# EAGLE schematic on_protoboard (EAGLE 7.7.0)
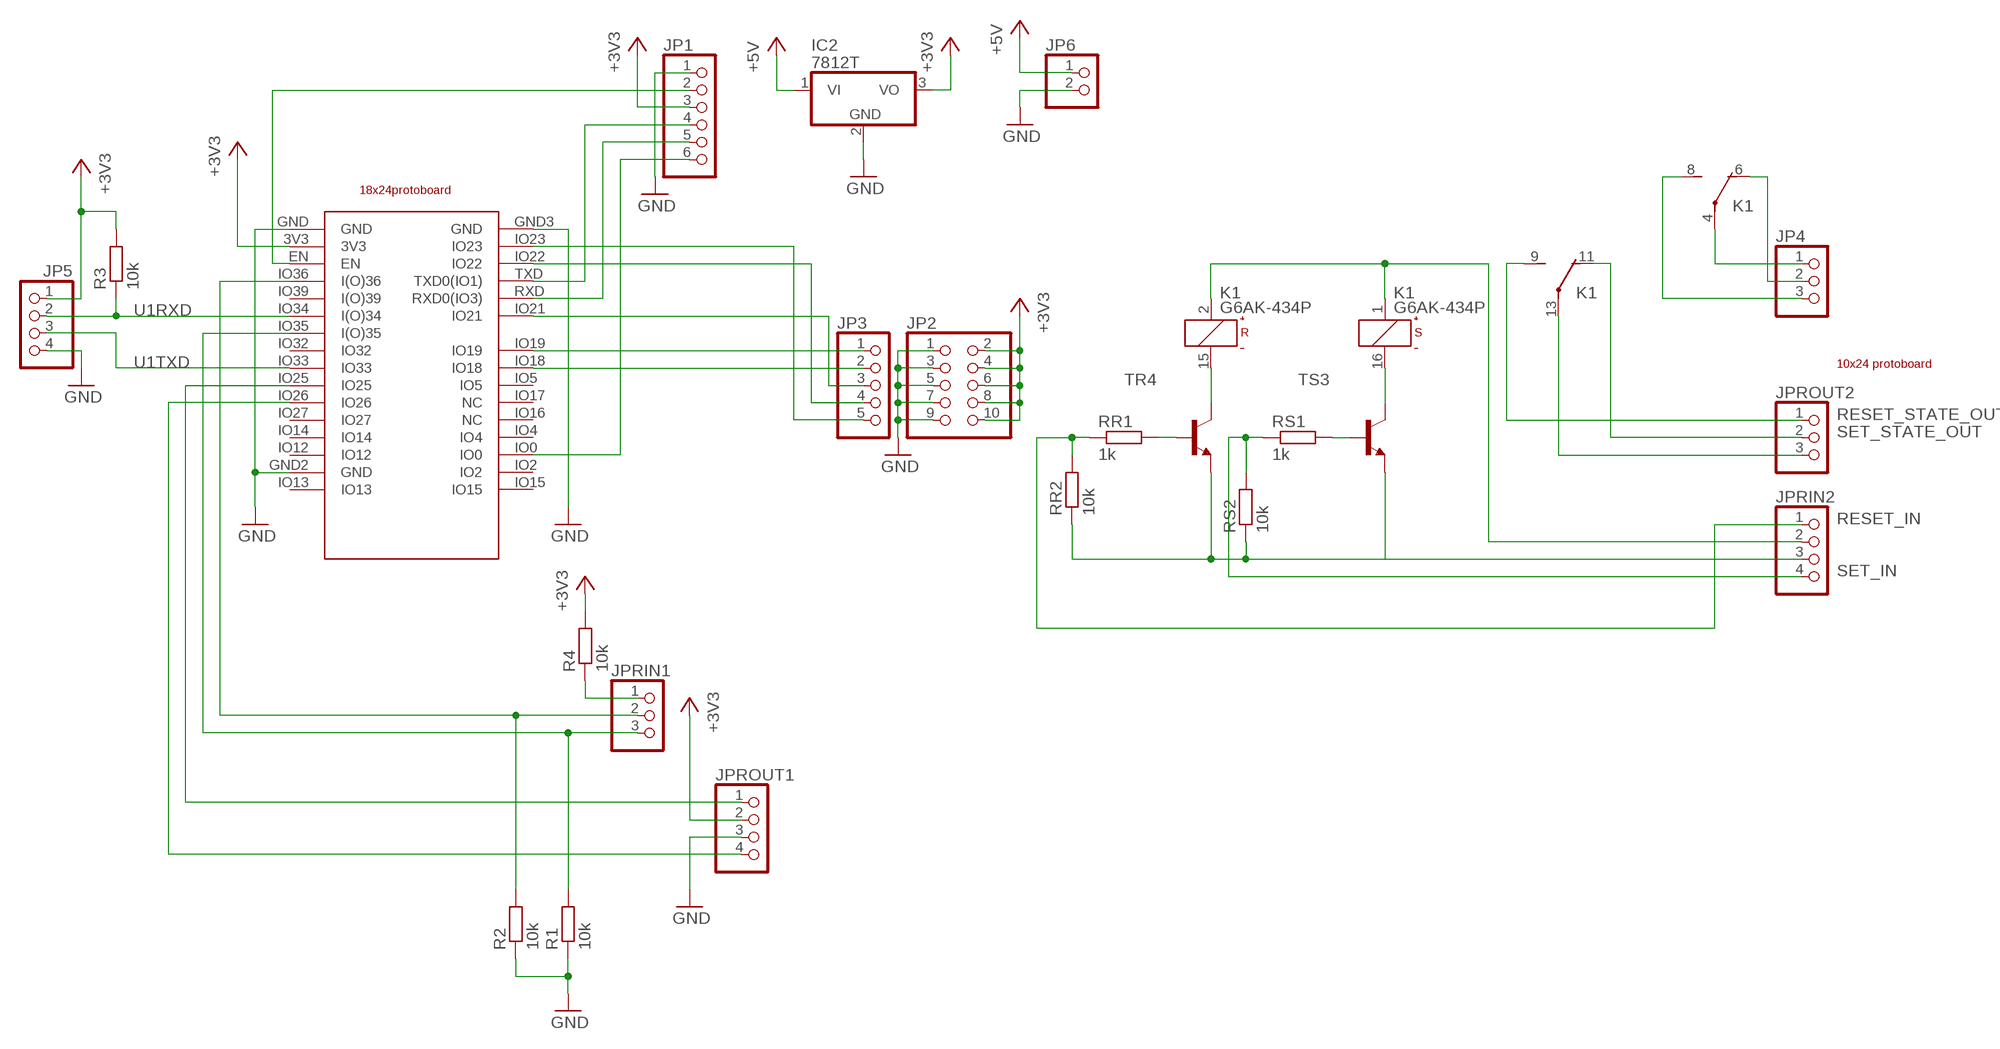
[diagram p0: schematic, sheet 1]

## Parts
ESP-32S-ADAPTER-PCB1  ESP-32S-ADAPTER-BREAKOUT  [ESP-32S-ADAPTER-PCB]
IC2  7812T  [TO220H]
JP1  PINHD-1X6/90  [1X06/90]
JP2  PINHD-2X5  [2X05]
JP3  PINHD-1X5  [1X05]
JP4  PINHD-1X3  [1X03]
JP5  PINHD-1X4  [1X04]
JP6  PINHD-1X2  [1X02]
JPRIN1  PINHD-1X3  [1X03]
JPRIN2  PINHD-1X4  [1X04]
JPROUT1  PINHD-1X4  [1X04]
JPROUT2  PINHD-1X3  [1X03]
K1  G6AK-434P  [G6AK-434P]
R1  10k  R-EU_R0603  [R0603]
R2  10k  R-EU_R0603  [R0603]
R3  10k  R-EU_R0603  [R0603]
R4  10k  R-EU_R0603  [R0603]
RR1  1k  R-EU_R0603  [R0603]
RR2  10k  R-EU_R0603  [R0603]
RS1  1k  R-EU_R0603  [R0603]
RS2  10k  R-EU_R0603  [R0603]
TR4  -NPN-TO92-EBC  [TO92-EBC]
TS3  -NPN-TO92-EBC  [TO92-EBC]
U$1  18X24  [PROTOBOARD_18X24_HOLE]
U$2  10X24  [PROTOBOARD_10X24_HOLE]

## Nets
+3V3: ESP-32S-ADAPTER-PCB1.3V3 IC2.3(VO) JP1.3 JP2.2 JP2.4 JP2.6 JP2.8 JP2.10 JP5.1 JPROUT1.2 R3.2 R4.2
+5V: IC2.1(VI) JP6.1
GND: ESP-32S-ADAPTER-PCB1.GND ESP-32S-ADAPTER-PCB1.GND2(GND) ESP-32S-ADAPTER-PCB1.GND3(GND) IC2.2(GND) JP1.1 JP2.1 JP2.3 JP2.5 JP2.7 JP2.9 JP5.4 JP6.2 JPROUT1.3 R1.1 R2.1
N$1: ESP-32S-ADAPTER-PCB1.EN JP1.2
N$2: JPRIN2.2 K1.1(-S:+) K1.2(-R:+)
N$3: ESP-32S-ADAPTER-PCB1.TXD(TXD0(IO1)) JP1.4
N$4: ESP-32S-ADAPTER-PCB1.RXD(RXD0(IO3)) JP1.5
N$5: K1.15(-R:-) TR4.C
N$6: ESP-32S-ADAPTER-PCB1.IO0 JP1.6
N$7: K1.16(-S:-) TS3.C
N$8: RS1.2 TS3.B
N$9: JPRIN2.3 RR2.1 RS2.1 TR4.E TS3.E
N$10: JPROUT2.3 K1.13(-2:P)
N$11: RR1.2 TR4.B
N$12: ESP-32S-ADAPTER-PCB1.IO19 JP3.1
N$13: ESP-32S-ADAPTER-PCB1.IO18 JP3.2
N$14: ESP-32S-ADAPTER-PCB1.IO21 JP3.3
N$15: JP4.1 K1.4(-1:P)
N$16: JP4.3 K1.8(-1:S)
N$17: ESP-32S-ADAPTER-PCB1.IO22 JP3.4
N$18: ESP-32S-ADAPTER-PCB1.IO35(I(O)35) JPRIN1.3 R1.2
N$19: JP4.2 K1.6(-1:O)
N$20: ESP-32S-ADAPTER-PCB1.IO36(I(O)36) JPRIN1.2 R2.2
N$21: ESP-32S-ADAPTER-PCB1.IO23 JP3.5
N$22: JPRIN1.1 R4.1
N$23: ESP-32S-ADAPTER-PCB1.IO25 JPROUT1.1
N$24: ESP-32S-ADAPTER-PCB1.IO26 JPROUT1.4
RESET_IN: JPRIN2.1 RR1.1 RR2.2
RESET_STATE_OUT: JPROUT2.1 K1.9(-2:S)
SET_IN: JPRIN2.4 RS1.1 RS2.2
SET_STATE_OUT: JPROUT2.2 K1.11(-2:O)
U1RXD: ESP-32S-ADAPTER-PCB1.IO34(I(O)34) JP5.2 R3.1
U1TXD: ESP-32S-ADAPTER-PCB1.IO33 JP5.3
Unconnected: ESP-32S-ADAPTER-PCB1.IO2 ESP-32S-ADAPTER-PCB1.IO4 ESP-32S-ADAPTER-PCB1.IO5 ESP-32S-ADAPTER-PCB1.IO12 ESP-32S-ADAPTER-PCB1.IO13 ESP-32S-ADAPTER-PCB1.IO14 ESP-32S-ADAPTER-PCB1.IO15 ESP-32S-ADAPTER-PCB1.IO16(NC) ESP-32S-ADAPTER-PCB1.IO17(NC) ESP-32S-ADAPTER-PCB1.IO27 ESP-32S-ADAPTER-PCB1.IO32 ESP-32S-ADAPTER-PCB1.IO39(I(O)39) K1.3(-4:P) K1.5(-4:O) K1.7(-4:S) K1.10(-3:S) K1.12(-3:O) K1.14(-3:P)

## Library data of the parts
ESP-32S-ADAPTER-PCB1 = ESP-32s-adapter-breakout:ESP-32S-ADAPTER-BREAKOUT
IC2 = linear:78*: Positive VOLTAGE REGULATOR Source: http://cache.national.com/ds/LM/LM78L05.pdf http://www.fairchildsemi.com/ds/LM/LM7805.pdf
JP1 = pinhead:PINHD-1X6: PIN HEADER
JP2 = pinhead:PINHD-2X5: PIN HEADER
JP3 = pinhead:PINHD-1X5: PIN HEADER
JP4 JPRIN1 JPROUT2 = pinhead:PINHD-1X3: PIN HEADER
JP5 JPRIN2 JPROUT1 = pinhead:PINHD-1X4: PIN HEADER
JP6 = pinhead:PINHD-1X2: PIN HEADER
K1 = relay:G6AK-434P: RELAY 4 x switch, dual coil latching, 0.3 A/125 V AC, 1 A/30 V DC, Omron; OC_FARNELL: unknown; OC_NEWARK: unknown
R1-R4 RR1 RR2 RS1 RS2 = rcl:R-EU_: RESISTOR, European symbol
TR4 TS3 = transistor:*-NPN-: NPN Transistror BF959 corrected 2008.03.06
U$1 = Protoboards:18X24
U$2 = Protoboards:10X24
